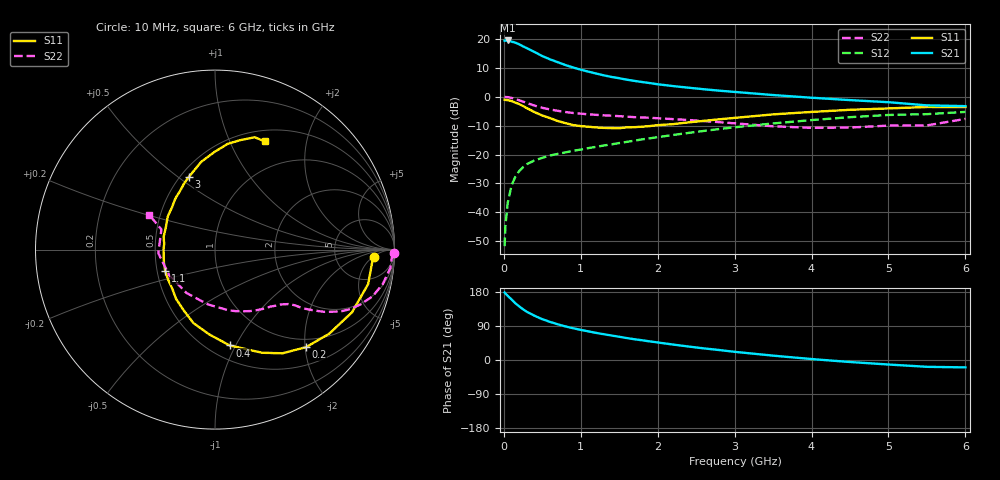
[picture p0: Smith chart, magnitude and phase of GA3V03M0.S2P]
! Infineon Technologies  Discrete & RF Semiconductors
! BF775
! Si NPN RF Bipolar Junction Transistor in SOT23
! VCE = 3 V  IC = 3 mA
! Common Emitter S-Parameters:  May  1996
# GHz  S  MA  R  50
!  f  S11  S21  S12  S22
! GHz  MAG  ANG  MAG  ANG  MAG  ANG  MAG  ANG
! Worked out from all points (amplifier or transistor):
!   36 points, 10 MHz to 6 GHz, reference 50 ohm
!   highest |S21| = 19.5 dB at 50 MHz (marker M1)
!   |S21| within 3 dB of that: start of sweep to 324 MHz
!   unconditionally stable (mu >= 1): 979.2 MHz to 3.687 GHz; 5.468 GHz to 5.559 GHz
!   at 250 MHz: K = 0.36, MSG = 20.9 dB, |S12| = -24.4 dB
!   at 1.4 GHz: K = 1.13, MAG = 9.5 dB, |S12| = -16.5 dB
!   at 6 GHz: K = 0.98, MSG = 1.0 dB, |S12| = -5.3 dB
!   S11 on the Smith chart (normalised r, x): 10 MHz: 15, -5; 200 MHz: 0.83, -2.02; 400 MHz: 0.63, -0.95; 1.1 GHz: 0.55, -0.15; 3 GHz: 0.55, +0.55; 6 GHz: 0.63, +1.36
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0.01  0.8862 -2.6  9.282 178.1  0.0026 85.3  0.9953 -1.2
0.02  0.8779 -5.0  9.346 175.6  0.0057 88.8  0.9868 -2.3
0.05  0.8746 -12.7  9.39 169.5  0.0145 83.5  0.9824 -6.0
0.1  0.8394 -24.6  8.97 159.8  0.0292 76.2  0.9542 -11.6
0.15  0.7902 -36.4  8.6 149.4  0.0415 69.9  0.915 -16.6
0.2  0.7433 -47.0  8.049 141.4  0.0518 65.3  0.8671 -20.6
0.25  0.6895 -56.9  7.412 133.8  0.0604 61.2  0.8223 -23.8
0.3  0.6323 -65.4  6.893 127.1  0.0683 58.3  0.779 -26.3
0.4  0.5402 -81.3  5.926 116.6  0.0792 53.7  0.7001 -29.7
0.5  0.4731 -94.0  5.045 107.7  0.0877 51.1  0.6419 -31.8
0.6  0.4265 -106.4  4.429 100.6  0.0961 49.7  0.6028 -33.2
0.7  0.38 -117.5  3.95 94.2  0.1025 49.3  0.57 -34.2
0.9  0.3227 -137.6  3.201 83.8  0.1157 49.4  0.5227 -35.7
1.1  0.3022 -156.5  2.709 75.5  0.1292 49.8  0.4959 -37.9
1.3  0.2882 -172.6  2.341 68.0  0.1433 50.3  0.4761 -40.0
1.6  0.2949 165.9  1.966 57.8  0.1658 50.7  0.4518 -44.2
2.2  0.3355 135.7  1.526 40.8  0.2178 49.7  0.4097 -55.4
3  0.4302 109.8  1.21 21.6  0.2957 44.0  0.3465 -77.5
3.5  0.4946 99.0  1.068 11.5  0.3449 38.8  0.3078 -97.4
4.5  0.5937 83.1  0.873 -5.3  0.4426 26.2  0.2925 -150.8
5.5  0.6639 70.5  0.708 -18.0  0.4992 10.9  0.3191 159.4
6  0.6631 65.4  0.687 -19.5  0.5458 6.6  0.4132 152.2
